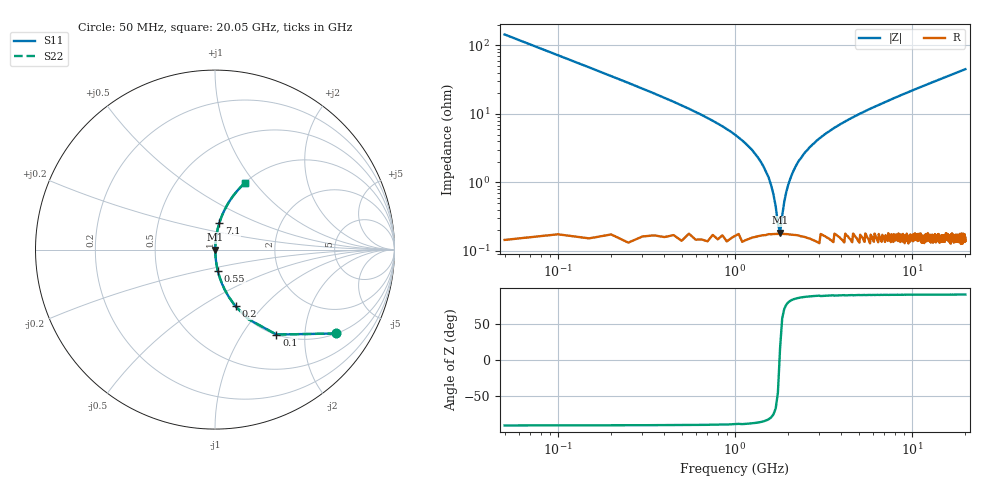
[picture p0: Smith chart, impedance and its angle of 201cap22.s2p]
! AVX Thin Film Operation		Date: May 2007
! Description: Accu-P® Series, Thin Film, SMD, RF Capacitor
! Part Number: 0201ZK220FBS
! 50 MHz  -  20.05 GHz
! Serial Measurements
# MHZ S MA R 50
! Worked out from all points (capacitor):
!   401 points, 50 MHz to 20.05 GHz, reference 50 ohm
!   read as one part in series: C = 22 pF near 150 MHz
!   lowest |Z| = 185 mohm at 1.8 GHz (marker M1)
!   series resonance near 1.788 GHz, so ESL is about 360 pH
!   S11 on the Smith chart (normalised r, x): 50 MHz: 1.00, -2.89; 100 MHz: 1.00, -1.44; 200 MHz: 1.00, -0.71; 550 MHz: 1.00, -0.24; 7.1 GHz: 1.00, +0.30; 20.05 GHz: 1.00, +0.90
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50  0.822 -34.7  0.569 55.3  0.569 55.3  0.822 -34.7
100  0.584 -54.1  0.81 35.8  0.81 35.8  0.584 -54.1
200  0.336 -70.1  0.94 19.6  0.94 19.6  0.336 -70.1
300  0.228 -76.5  0.972 13.2  0.972 13.2  0.228 -76.5
550  0.118 -82.5  0.991 6.8  0.991 6.8  0.118 -82.5
1350  0.023 -84.8  0.998 1.3  0.998 1.3  0.023 -84.8
1550  0.012 -81.7  0.998 0.7  0.998 0.7  0.012 -81.7
1700  0.004378 -69.1  0.998 0.2  0.998 0.2  0.004378 -69.1
1750  0.002338 -48.4  0.998 0.1  0.998 0.1  0.002338 -48.4
1800  0.001634 18.7  0.998 -0.0  0.998 -0.0  0.001634 18.7
1850  0.003145 60.4  0.998 -0.2  0.998 -0.2  0.003145 60.4
2050  0.011 81.4  0.998 -0.6  0.998 -0.6  0.011 81.4
2300  0.021 84.5  0.998 -1.2  0.998 -1.2  0.021 84.5
2750  0.036 85.5  0.998 -2.1  0.998 -2.1  0.036 85.5
3400  0.055 85.2  0.997 -3.2  0.997 -3.2  0.055 85.2
4650  0.089 83.9  0.994 -5.1  0.994 -5.1  0.089 83.9
6750  0.14 81.3  0.989 -8.1  0.989 -8.1  0.14 81.3
7100  0.149 80.9  0.987 -8.5  0.987 -8.5  0.149 80.9
10050  0.215 77.2  0.975 -12.4  0.975 -12.4  0.215 77.2
13400  0.285 73.1  0.957 -16.6  0.957 -16.6  0.285 73.1
16750  0.35 69.3  0.935 -20.5  0.935 -20.5  0.35 69.3
20050  0.41 65.6  0.911 -24.2  0.911 -24.2  0.41 65.6
